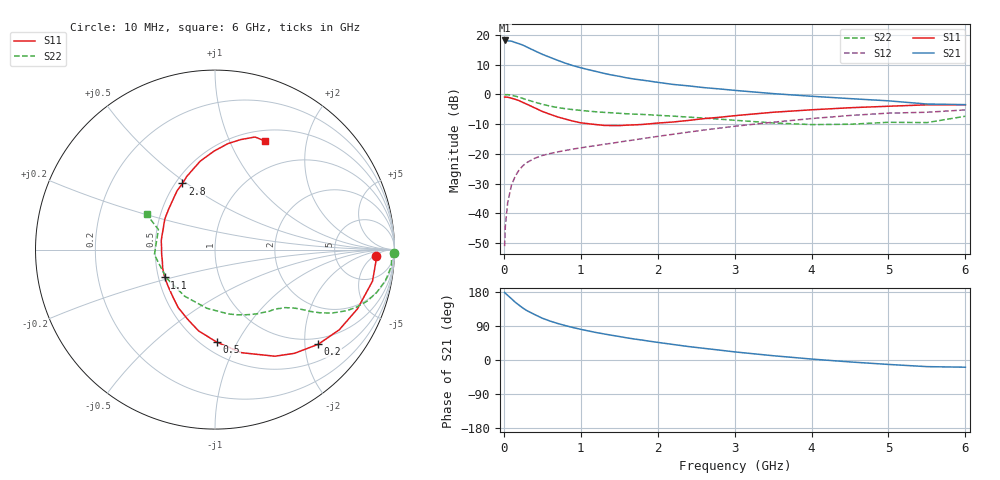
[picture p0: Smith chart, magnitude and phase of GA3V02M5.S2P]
! Infineon Technologies  Discrete & RF Semiconductors
! BF775
! Si NPN RF Bipolar Junction Transistor in SOT23
! VCE = 3 V  IC = 2.5 mA
! Common Emitter S-Parameters:  May  1996
# GHz  S  MA  R  50
!  f  S11  S21  S12  S22
! GHz  MAG  ANG  MAG  ANG  MAG  ANG  MAG  ANG
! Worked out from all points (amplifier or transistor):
!   36 points, 10 MHz to 6 GHz, reference 50 ohm
!   highest |S21| = 18.1 dB at 10 MHz (marker M1)
!   |S21| within 3 dB of that: start of sweep to 362.9 MHz
!   unconditionally stable (mu >= 1): 1.077 GHz to 3.809 GHz; 5.374 GHz to 5.704 GHz
!   at 250 MHz: K = 0.32, MSG = 20.2 dB, |S12| = -24.0 dB
!   at 1.4 GHz: K = 1.12, MAG = 9.4 dB, |S12| = -16.5 dB
!   at 6 GHz: K = 0.98, MSG = 0.9 dB, |S12| = -5.2 dB
!   S11 on the Smith chart (normalised r, x): 10 MHz: 16, -6; 200 MHz: 0.85, -2.30; 500 MHz: 0.59, -0.83; 1.1 GHz: 0.54, -0.19; 2.8 GHz: 0.54, +0.48; 6 GHz: 0.62, +1.36
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0.01  0.8993 -2.4  8.046 178.3  0.0028 88.4  0.9966 -1.0
0.02  0.8983 -4.6  7.97 176.1  0.0062 87.0  0.9844 -2.1
0.05  0.8951 -11.3  7.928 170.6  0.0151 83.3  0.9872 -5.3
0.1  0.8597 -22.6  7.828 161.5  0.03 77.7  0.9655 -10.3
0.15  0.824 -32.8  7.415 152.2  0.0425 71.2  0.9309 -15.0
0.2  0.7806 -42.5  7.078 144.4  0.0538 66.9  0.8939 -18.8
0.25  0.7278 -52.6  6.695 136.7  0.0634 62.3  0.8504 -22.2
0.3  0.6811 -60.7  6.23 130.3  0.0713 59.0  0.8087 -24.9
0.4  0.5931 -75.6  5.403 120.0  0.084 54.0  0.7394 -28.6
0.5  0.5161 -88.8  4.708 110.3  0.0938 50.6  0.6808 -31.1
0.6  0.4618 -101.5  4.184 102.8  0.1009 48.6  0.6342 -32.9
0.7  0.4167 -111.5  3.727 96.4  0.1076 47.5  0.5996 -34.1
0.9  0.3544 -131.1  3.033 85.6  0.1203 46.6  0.5529 -36.2
1.1  0.3204 -151.1  2.598 76.7  0.1319 47.0  0.5219 -38.4
1.3  0.3004 -167.5  2.254 68.9  0.1443 47.6  0.4975 -40.7
1.6  0.3035 170.5  1.888 58.4  0.1647 48.4  0.4707 -44.9
2.2  0.3425 139.0  1.467 41.0  0.2132 48.4  0.43 -56.1
2.8  0.4106 116.2  1.233 26.2  0.27 45.3  0.3827 -71.5
3.5  0.4996 99.5  1.028 11.3  0.3398 38.9  0.3302 -97.8
4.5  0.5951 83.0  0.847 -5.1  0.4409 26.6  0.3139 -150.0
5.5  0.6658 70.4  0.687 -17.5  0.4996 11.0  0.3346 160.4
6  0.666 65.5  0.671 -19.0  0.5466 6.6  0.4285 152.8
